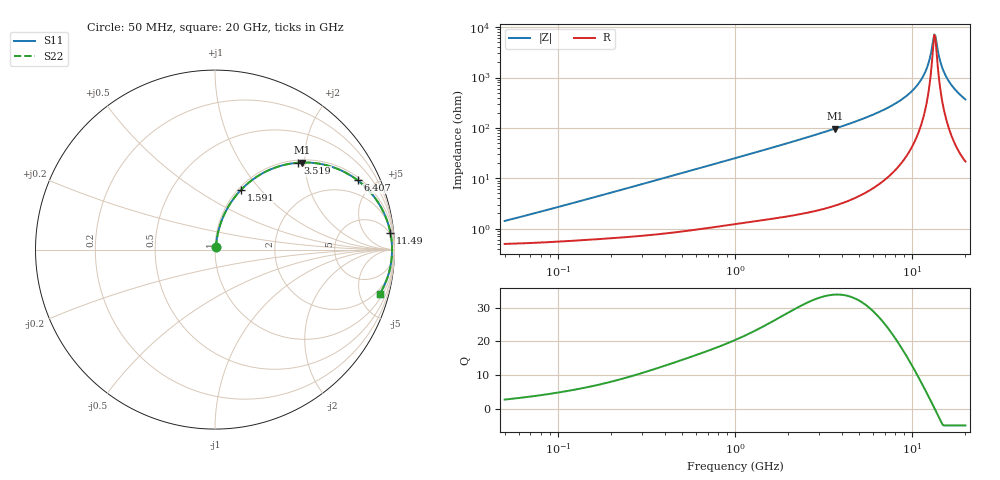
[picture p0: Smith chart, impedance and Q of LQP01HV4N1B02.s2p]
!Murata Part Number: LQP01HV4N1B02
!These Parameters are Measured in Series Mode Connection
!  o--[Z]--o
!Port1  Port2
!  o-------o
!Freq. Start=50[MHz] Stop=20[GHz], 401[Steps]
# Hz S RI R 50
!Freq.(Hz) S11(Real) S11(Imag) S21(Real) S21(Imag) S12(Real) S12(Imag) S22(Real) S22(Imag)
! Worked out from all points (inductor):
!   401 points, 50 MHz to 20 GHz, reference 50 ohm
!   read as one part in series: L = 4.22 nH near 57.22 MHz
!   highest Q = 33.8 at 3.681 GHz (marker M1), where L = 4.2 nH
!   self-resonance near 13.35 GHz
!   S11 on the Smith chart (normalised r, x): 50 MHz: 1.01, +0.03; 1.591 GHz: 1.03, +0.80; 3.519 GHz: 1.05, +1.85; 6.407 GHz: 1.15, +4.03; 11.49 GHz: 4, +20; 20 GHz: 1.43, -7.33
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5e7  0.00513 0.0132  0.9949 -0.0132  0.9949 -0.0132  0.00513 0.0132
1.364002e8  0.0071 0.0351  0.9929 -0.0351  0.9929 -0.0351  0.0071 0.0351
3.721004e8  0.0164 0.0923  0.9836 -0.0923  0.9836 -0.0923  0.0164 0.0923
1e9  0.0689 0.23  0.9311 -0.23  0.9311 -0.23  0.0689 0.23
1.590961e9  0.1462 0.3343  0.8538 -0.3343  0.8538 -0.3343  0.1462 0.3343
2.728004e9  0.3318 0.4556  0.6682 -0.4556  0.6682 -0.4556  0.3318 0.4556
3.519108e9  0.4614 0.4839  0.5386 -0.4839  0.5386 -0.4839  0.4614 0.4839
3.680849e9  0.4864 0.4853  0.5136 -0.4853  0.5136 -0.4853  0.4864 0.4853
4.81993e9  0.6412 0.4645  0.3588 -0.4645  0.3588 -0.4645  0.6412 0.4645
6.406762e9  0.7943 0.3865  0.2057 -0.3865  0.2057 -0.3865  0.7943 0.3865
7.442007e9  0.8615 0.3247  0.1385 -0.3247  0.1385 -0.3247  0.8615 0.3247
9.745021e9  0.9486 0.1875  0.0514 -0.1875  0.0514 -0.1875  0.9486 0.1875
1.066139e10  0.9667 0.1366  0.0333 -0.1366  0.0333 -0.1366  0.9667 0.1366
1.149051e10  0.9774 0.0929  0.0226 -0.0929  0.0226 -0.0929  0.9774 0.0929
1.238412e10  0.9841 0.0482  0.0159 -0.0482  0.0159 -0.0482  0.9841 0.0482
1.314879e10  0.9864 0.012  0.0136 -0.012  0.0136 -0.012  0.9864 0.012
1.354865e10  0.9865 -0.00619  0.0135 0.00619  0.0135 0.00619  0.9865 -0.00619
1.375312e10  0.9863 -0.0153  0.0137 0.0153  0.0137 0.0153  0.9863 -0.0153
1.460232e10  0.9838 -0.052  0.0162 0.052  0.0162 0.052  0.9838 -0.052
1.550395e10  0.9784 -0.0888  0.0216 0.0888  0.0216 0.0888  0.9784 -0.0888
1.721783e10  0.9616 -0.1534  0.0384 0.1534  0.0384 0.1534  0.9616 -0.1534
2e10  0.9183 -0.2459  0.0817 0.2459  0.0817 0.2459  0.9183 -0.2459
